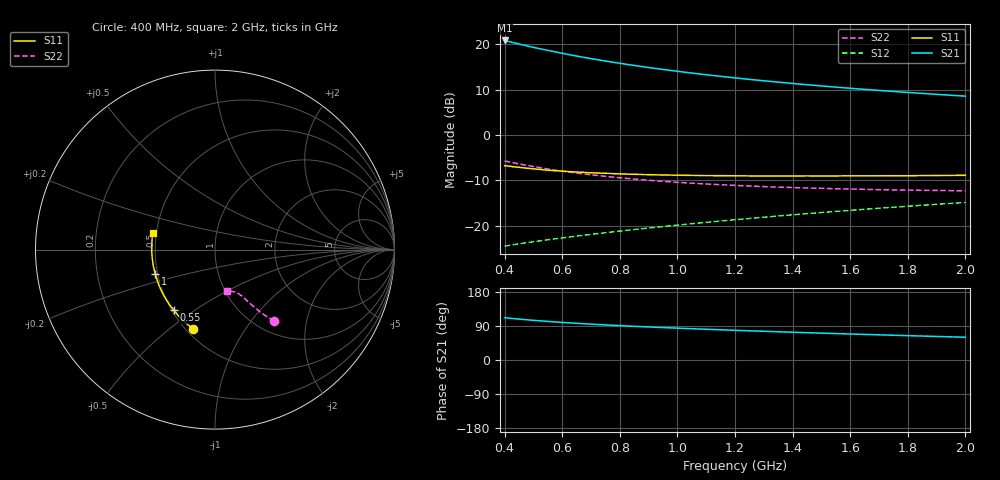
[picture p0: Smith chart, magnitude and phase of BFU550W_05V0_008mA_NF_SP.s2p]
! Filename:  P:\Prog\Test\Noise\ATS_data\Testdata_Net\06 Compressed Noise after Statistics\BFU550W_APM2013_11_D05_05p0V_008mA_NF_CM01_D.sf
! Date/Time: Tue 26/Mar/2013 16:25:22
! BFU550W_APM2013_11_D05_05p0V_1to35mA_NF_CM01_Bias5_R.sf
! Noise Parameter Data File
! BFU550W_APM2013_11_D05_05p0V_1to35mA_NF_CM01
! Date/time: Mon Mar 25 13:26:50 2013
! VAR V_out= 5.000000
! VAR I_out= 7.995000
! VAR V_in= 0.818800
! VAR I_in= 0.082805
! Device data file deembeded for feedlines and parallel
! Original file: \06 Compressed Noise after Statistics\BFU550W_APM2013_11_D05_05p0V_008mA_NF_CM01_R.sf
! Feed-files: PR019V01_070313_Feed1.s2p, PR019V01_070313_Feed2.s2p
! Parallel-file: PR019V01_070313_Par.s2p
# MHz S MA R 50
!  Freq-MHz  S11-mag  S11-arg  S21-mag  S21-arg  S12-mag  S12-arg  S22-mag  S22-arg
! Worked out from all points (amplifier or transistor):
!   37 points, 400 MHz to 2 GHz, reference 50 ohm
!   highest |S21| = 20.9 dB at 400 MHz (marker M1)
!   |S21| within 3 dB of that: start of sweep to 613.6 MHz
!   unconditionally stable (mu >= 1): 1.491 GHz to end of sweep
!   at 500 MHz: K = 0.67, MSG = 21.5 dB, |S12| = -23.6 dB
!   at 1.1 GHz: K = 0.95, MSG = 16.3 dB, |S12| = -19.3 dB
!   at 2 GHz: K = 1.02, MAG = 10.9 dB, |S12| = -14.9 dB
!   lowest NFmin = 0.64 dB at 420 MHz
!   S11 on the Smith chart (normalised r, x): 400 MHz: 0.54, -0.61; 550 MHz: 0.51, -0.42; 1 GHz: 0.48, -0.15; 2 GHz: 0.48, +0.10
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400  0.4586 -105.2  11.05 111.6  0.05916 56.2  0.5156 -50.2
420  0.45 -108.0  10.65 110.1  0.06069 56.0  0.5006 -50.9
440  0.4425 -110.8  10.27 108.6  0.06213 55.9  0.486 -51.6
460  0.4356 -113.4  9.916 107.3  0.06349 55.9  0.4725 -52.2
500  0.4226 -118.6  9.269 104.7  0.06625 55.9  0.448 -53.3
550  0.4081 -124.1  8.585 101.8  0.06963 56.2  0.421 -54.4
600  0.3987 -129.3  7.973 99.2  0.07306 56.5  0.3981 -55.2
650  0.3896 -133.8  7.436 96.8  0.07647 56.8  0.3799 -56.0
700  0.3826 -138.2  6.967 94.6  0.07986 57.2  0.3632 -56.7
750  0.3771 -142.1  6.552 92.6  0.08329 57.7  0.3488 -57.3
800  0.3715 -145.9  6.182 90.7  0.0868 58.1  0.337 -58.0
850  0.3679 -149.4  5.853 88.9  0.09026 58.5  0.3255 -58.4
950  0.3612 -155.3  5.288 85.6  0.09743 59.2  0.3076 -59.4
1000  0.3597 -158.2  5.047 84.1  0.101 59.5  0.2998 -59.8
1100  0.356 -163.2  4.623 81.1  0.1084 60.1  0.2876 -61.0
1200  0.354 -167.9  4.269 78.4  0.1159 60.5  0.2776 -62.2
1250  0.353 -170.3  4.109 77.0  0.1197 60.7  0.273 -62.6
1350  0.3525 -174.2  3.83 74.5  0.1274 61.0  0.2654 -63.8
1500  0.3523 -179.9  3.477 70.9  0.1391 61.2  0.2574 -65.9
1650  0.3533 175.0  3.187 67.5  0.1511 61.2  0.2509 -68.0
1750  0.3547 172.0  3.024 65.3  0.1592 61.2  0.247 -69.6
2000  0.3587 164.7  2.683 60.1  0.1797 60.6  0.2418 -74.0
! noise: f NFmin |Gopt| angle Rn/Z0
400  0.6606  0.05751  114.5  0.0806
460  0.661  0.07562  118.3  0.08
600  0.6996  0.0882  124  0.0813
800  0.7227  0.1352  136.7  0.073
1000  0.7528  0.17  145.3  0.0677
1200  0.805  0.1924  152.9  0.0667
1400  0.8261  0.2316  162.7  0.0625
1600  0.8268  0.2559  166.4  0.0618
1800  0.8957  0.2964  -178.6  0.0543
2000  0.9226  0.3261  -172.1  0.0525
